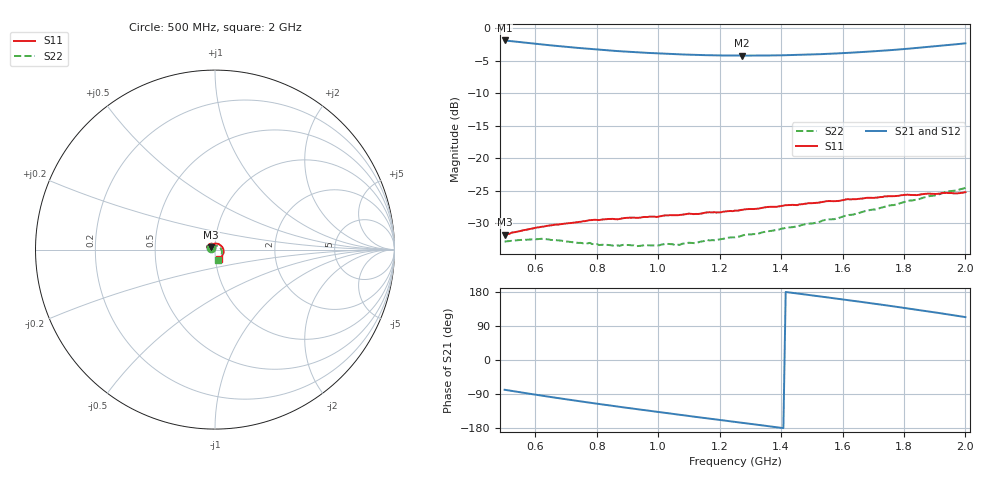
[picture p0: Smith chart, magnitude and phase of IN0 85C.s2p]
!Agilent Technologies,E8363B,SG43030131,A.07.50.48
!Agilent E8363B: A.07.50.48
!Date: Friday, October 17, 2025 03:42:32
!Correction: S11(Full 2 Port(1,2))
!S21(Full 2 Port(1,2))
!S12(Full 2 Port(1,2))
!S22(Full 2 Port(1,2))
!S2P File: Measurements: S11, S21, S12, S22:
# Hz S  dB  R 50
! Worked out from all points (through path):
!   201 points, 500 MHz to 2 GHz, reference 50 ohm
!   highest |S21| = -1.91 dB at 500 MHz (marker M1); lowest = -4.2 dB at 1.272 GHz (marker M2)
!   group delay of S21, straight-line fit = 302 ps
!   lowest |S11| = -31.7 dB at 500 MHz (marker M3), VSWR 1.05, Z = 47.9 + j1.38 ohm
!   |S11| at or under -10 dB: start of sweep to end of sweep
!   |S22| runs from -33.5 to -24.6 dB; largest |S21 - S12| = 0.0013
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5e8  -31.75 146.2  -1.91 -78.5  -1.91 -78.6  -32.80 153.5
6.2e8  -30.52 121.5  -2.52 -93.9  -2.52 -94.0  -32.37 132.8
7.55e8  -29.69 97.5  -3.12 -110.1  -3.13 -110.1  -33.06 114.7
7.775e8  -29.51 93.8  -3.21 -112.7  -3.21 -112.7  -33.00 111.4
8.075e8  -29.50 89.5  -3.32 -116.1  -3.33 -116.1  -33.34 107.6
8.6e8  -29.36 82.2  -3.51 -122.0  -3.51 -122.0  -33.49 99.3
8.825e8  -29.25 79.1  -3.58 -124.5  -3.59 -124.5  -33.33 97.6
1.0025e9  -28.96 63.7  -3.90 -137.5  -3.92 -137.5  -33.40 83.3
1.025e9  -28.78 60.7  -3.96 -139.9  -3.96 -139.9  -33.16 80.7
1.055e9  -28.74 57.2  -4.02 -143.1  -4.02 -143.1  -33.36 76.6
1.1e9  -28.51 52.0  -4.09 -147.8  -4.09 -147.8  -32.98 70.7
1.1225e9  -28.55 49.4  -4.12 -150.1  -4.13 -150.2  -33.06 68.4
1.16e9  -28.32 45.3  -4.16 -154.1  -4.17 -154.1  -32.57 64.0
1.19e9  -28.34 41.9  -4.20 -157.2  -4.20 -157.2  -32.57 60.1
1.25e9  -28.04 35.0  -4.23 -163.4  -4.23 -163.4  -32.14 52.0
1.2725e9  -27.93 32.7  -4.24 -165.7  -4.24 -165.7  -31.90 49.6
1.3775e9  -27.47 20.9  -4.20 -176.6  -4.21 -176.6  -31.07 34.3
1.505e9  -26.89 6.7  -4.05 170.1  -4.06 170.1  -30.00 15.1
1.6325e9  -26.31 -8.6  -3.77 156.4  -3.78 156.4  -28.68 -6.6
1.7525e9  -25.84 -25.2  -3.41 143.1  -3.40 143.0  -27.26 -27.7
1.88e9  -25.44 -45.5  -2.90 128.1  -2.90 128.1  -25.85 -51.5
2e9  -25.21 -68.8  -2.35 113.2  -2.35 113.1  -24.56 -75.2
